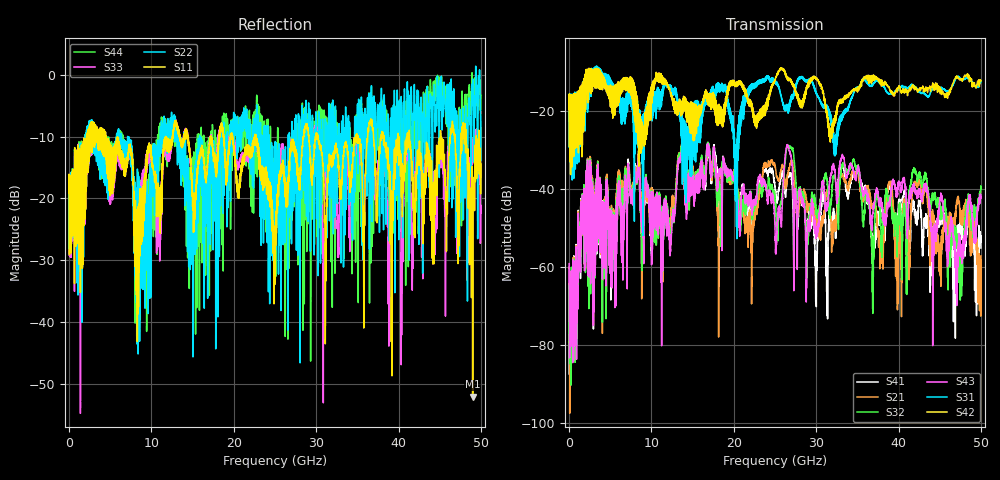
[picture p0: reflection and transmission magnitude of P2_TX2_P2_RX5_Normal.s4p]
!Keysight Technologies,N5225B,MY57041031,A.13.20.10
!Date: Friday, May 31, 2019 11:34:12
!Correction: S11(Full 4 Port(1,2,3,4))
!S12(Full 4 Port(1,2,3,4))
!S13(Full 4 Port(1,2,3,4))
!S14(Full 4 Port(1,2,3,4))
!S21(Full 4 Port(1,2,3,4))
!S22(Full 4 Port(1,2,3,4))
!S23(Full 4 Port(1,2,3,4))
!S24(Full 4 Port(1,2,3,4))
!S31(Full 4 Port(1,2,3,4))
!S32(Full 4 Port(1,2,3,4))
!S33(Full 4 Port(1,2,3,4))
!S34(Full 4 Port(1,2,3,4))
!S41(Full 4 Port(1,2,3,4))
!S42(Full 4 Port(1,2,3,4))
!S43(Full 4 Port(1,2,3,4))
!S44(Full 4 Port(1,2,3,4))
!S4P File: Measurements: <S11,S12,S13,S14>,
!<S21,S22,S23,S24>,
!<S31,S32,S33,S34>,
!<S41,S42,S43,S44>:
# Hz S  dB  R 50.0
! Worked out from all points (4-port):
!   5000 points, 10 MHz to 50 GHz, reference 50 ohm
!   strongest paths, dB at 10 MHz, 12.51 GHz, 25.01 GHz, 37.51 GHz, 50 GHz:
!     S42: -19.5, -16.9, -12.1, -11.6, -12.3
!     S31: -19.4, -14.8, -13.0, -12.4, -12.6
!     S43: -59.1, -48.3, -51.0, -40.8, -42.0
!     S32: -64.7, -46.9, -43.8, -42.5, -40.0
!     S21: -60.0, -43.0, -34.1, -50.5, -57.2
!     S41: -66.3, -44.6, -39.5, -47.8, -55.1
!   lowest |S11| = -52.1 dB at 49 GHz (marker M1), VSWR 1.00, Z = 49.8 + j0.0602 ohm
!   |S11| at or under -10 dB: 4.481 GHz to 11.72 GHz (7.238 GHz wide, 89.4 % of centre); 22.73 GHz to 28.47 GHz (5.744 GHz wide, 22.4 % of centre); 30.26 GHz to 34.82 GHz (4.562 GHz wide, 14 % of centre)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
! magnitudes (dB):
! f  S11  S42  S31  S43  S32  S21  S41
! 10 MHz  -19.1  -19.5  -19.4  -59.1  -64.7  -60.0  -66.3
! 2.3 GHz  -15.8  -17.9  -19.4  -36.5  -36.3  -36.0  -36.2
! 12.25 GHz  -10.7  -14.8  -13.4  -53.5  -52.1  -50.8  -51.0
! 13.65 GHz  -10.7  -19.2  -22.4  -30.5  -29.4  -29.2  -30.4
! 21.99 GHz  -13.3  -17.2  -13.8  -41.8  -42.9  -49.5  -47.0
! 49 GHz  -52.1  -13.0  -12.7  -48.2  -48.8  -52.1  -54.4
! 50 GHz  -14.4  -12.3  -12.6  -42.0  -40.0  -57.2  -55.1
